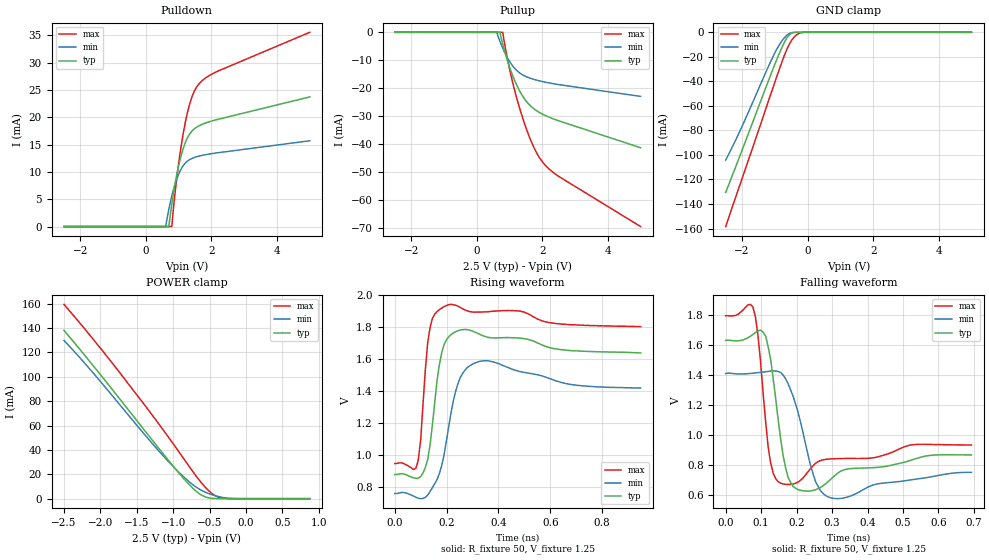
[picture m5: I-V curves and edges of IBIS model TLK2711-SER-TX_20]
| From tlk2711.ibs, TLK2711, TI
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|   Model TLK2711-SER-TX_20
[Model]   TLK2711-SER-TX_20
Model_type   3-state
Polarity   Non-Inverting
Enable   Active-Low
| Timing test load is based on data sheet information for rise and fall time
Vmeas = 1.5V
Cref  = 12.5pF
Rref  = 1Mohms
Vref  = 0V
| C_comp is estimated by modeling group by simulation
C_comp   0.9360pF   0.8158pF   0.9617pF
[Temperature Range]   27   85   -40
[Voltage Range]   2.5V   2.3V   2.7V
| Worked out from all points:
|   GND clamp passes 1 mA (typ) near -0.50 V on its own axis
|   POWER clamp passes 1 mA (typ) near -0.54 V on its own axis
|   rising waveform, R_fixture 50, V_fixture 1.25: 20-80 % time 32.2ps typ, 46.4ps min, 22.3ps max; typ from 0.878 V to 1.64 V
|   falling waveform, R_fixture 50, V_fixture 1.25: 20-80 % time 24.2ps typ, 43.9ps min, 19.3ps max; typ from 1.63 V to 0.864 V
[Pulldown]
| voltage   I(typ)   I(min)   I(max)
-2.5V     0A         0A         0A
600mV     5.79pA     2.02uA     0A
700mV     56.98uA    3.184mA    800fA
790mV     4.132mA    5.612mA    36.42uA
875mV     7.35mA     7.496mA    5.396mA
960mV     10.06mA    9.016mA    9.741mA
1.15V     14.49mA    11.26mA    17.44mA
1.325V    16.86mA    12.23mA    22.25mA
1.55V     18.21mA    12.79mA    25.58mA
1.775V    18.87mA    13.11mA    27.01mA
2.15V     19.56mA    13.48mA    28.33mA
5V        23.74mA    15.71mA    35.57mA
[Pullup]
| voltage   I(typ)   I(min)   I(max)
-2.5V     22.17nA    4.736uA    453.2nA
610mV     -23.82nA   -983.9nA   -32.1nA
710mV     -26.89uA   -3.333mA   -36.43nA
790mV     -4.097mA   -5.618mA   -2.251uA
900mV     -8.716mA   -8.355mA   -7.351mA
1.04V     -13.76mA   -11.13mA   -15.22mA
1.31V     -21.06mA   -14.57mA   -27.29mA
1.625V    -26.2mA    -16.43mA   -38.1mA
1.925V    -28.82mA   -17.44mA   -45.16mA
2.15V     -30.14mA   -18.01mA   -48.4mA
2.44V     -31.49mA   -18.62mA   -51.19mA
5V        -41.39mA   -22.98mA   -69.66mA
[GND_clamp]
| voltage   I(typ)   I(min)   I(max)
-2.5V     -130.6mA   -104.2mA   -158.4mA
-2.05V    -99.66mA   -79.61mA   -123.2mA
-1.225V   -41.59mA   -29.64mA   -58.49mA
-925mV    -21.19mA   -13.02mA   -34.91mA
-775mV    -11.89mA   -6.69mA    -23.59mA
-625mV    -4.281mA   -2.194mA   -13.44mA
-550mV    -1.797mA   -853.7uA   -9.328mA
-475mV    -515.9uA   -225.4uA   -6.047mA
-325mV    -16.34uA   -6.464uA   -1.843mA
-175mV    -335.2nA   -108.9nA   -179.3uA
-25mV     -17.29nA   -11.4nA    -5.392uA
5V        85.07nA    86.67nA    83.48nA
[POWER_clamp]
| voltage   I(typ)   I(min)   I(max)
-2.5V     138.1mA    129.8mA    159.4mA
-2.2V     116.5mA    110.1mA    138.2mA
-1.75V    83.01mA    78.25mA    104.6mA
-1.3V     48.95mA    46.12mA    69.52mA
-1V       26.62mA    26.3mA     44.98mA
-850mV    16.09mA    17.49mA    32.3mA
-700mV    6.829mA    10.06mA    19.69mA
-625mV    3.337mA    7.198mA    13.82mA
-475mV    282.6uA    3.358mA    4.459mA
-400mV    52.34uA    2.028mA    1.614mA
-250mV    1.171uA    360.3uA    76.11uA
875mV     0A         0A         0A
[Ramp]
| variable   typ   min   max
dV/dt_r 0.45018V/0.03132ns  0.39252V/0.0457867ns  0.50184V/0.0206132ns
dV/dt_f 0.44958V/0.0233656ns  0.3906V/0.0435273ns  0.50154V/0.0185225ns
R_load = 50
[Rising Waveform]
R_fixture = 50
V_fixture = 1.25
V_fixture_min = 1.00
V_fixture_max = 1.40
| time   V(typ)   V(min)   V(max)
0s        877.7mV    758.8mV    946.6mV
81ps      853.8mV    736mV      916mV
100ps     865.5mV    726.5mV    1.098V
118ps     922.5mV    734.9mV    1.539V
145ps     1.188V     795.1mV    1.856V
163ps     1.466V     846.5mV    1.899V
190ps     1.692V     999.9mV    1.93V
244ps     1.779V     1.449V     1.933V
325ps     1.759V     1.586V     1.896V
949ps     1.64V      1.42V      1.805V
[Falling Waveform]
R_fixture = 50
V_fixture = 1.25
V_fixture_min = 1.00
V_fixture_max = 1.40
| time   V(typ)   V(min)   V(max)
0s        1.628V     1.407V     1.792V
77ps      1.668V     1.409V     1.85V
91ps      1.691V     1.413V     1.664V
113ps     1.655V     1.419V     1.08V
127ps     1.499V     1.423V     809.9mV
155ps     972.2mV    1.414V     675.4mV
190ps     654mV      1.256V     670.2mV
253ps     631.8mV    689.6mV    807.1mV
288ps     684.3mV    585.1mV    836.1mV
693ps     864.1mV    748.3mV    930.4mV
